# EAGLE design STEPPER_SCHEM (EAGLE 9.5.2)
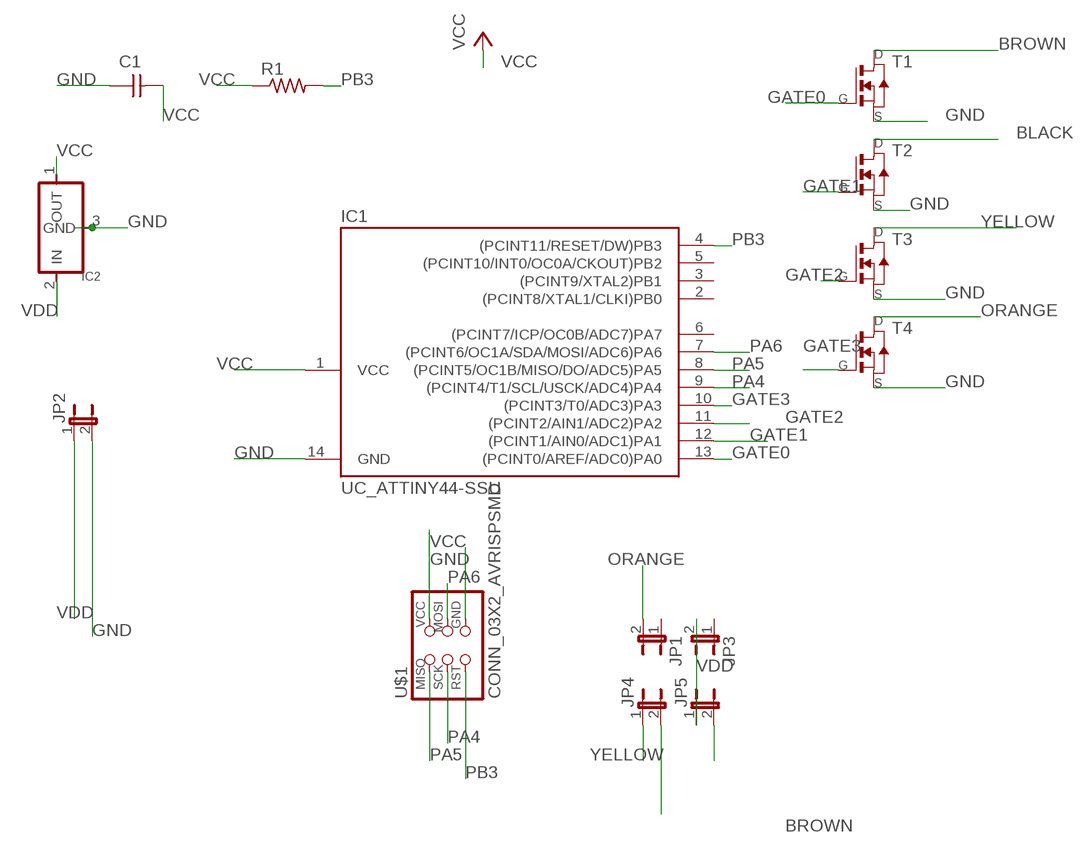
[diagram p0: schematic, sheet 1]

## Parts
C1  CAP_UNPOLARIZEDFAB  [C1206FAB]
IC1  UC_ATTINY44-SSU  [SOIC14]
IC2  VR_REGULATOR-SOT23SOT23  [SOT23]
JP1  JP1E  [JP1]
JP2  JP1E  [JP1]
JP3  JP1E  [JP1]
JP4  JP1E  [JP1]
JP5  JP1E  [JP1]
R1  R1206FAB  [R1206FAB]
T1  MOSFET_NSOT23  [SOT-23]
T2  MOSFET_NSOT23  [SOT-23]
T3  MOSFET_NSOT23  [SOT-23]
T4  MOSFET_NSOT23  [SOT-23]
U$1  CONN_03X2_AVRISPSMD  [2X03SMD]

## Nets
BLACK: JP4.2 T2.1(D)
BROWN: JP5.2 T1.1(D)
GATE0: IC1.13((PCINT0/AREF/ADC0)PA0) T1.3(G)
GATE1: IC1.12((PCINT1/AIN0/ADC1)PA1) T2.3(G)
GATE2: IC1.11((PCINT2/AIN1/ADC2)PA2) T3.3(G)
GATE3: IC1.10((PCINT3/T0/ADC3)PA3) T4.3(G)
GND: C1.1 IC1.14(GND) IC2.3(GND) JP2.2 T1.2(S) T2.2(S) T3.2(S) T4.2(S) U$1.6(GND)
ORANGE: JP1.2 T4.1(D)
PA4: IC1.9((PCINT4/T1/SCL/USCK/ADC4)PA4) U$1.3(SCK)
PA5: IC1.8((PCINT5/OC1B/MISO/DO/ADC5)PA5) U$1.1(MISO)
PA6: IC1.7((PCINT6/OC1A/SDA/MOSI/ADC6)PA6) U$1.4(MOSI)
PB3: IC1.4((PCINT11/RESET/DW)PB3) R1.2 U$1.5(RST)
VCC: C1.2 IC1.1(VCC) IC2.1(OUT) R1.1 U$1.2(VCC)
VDD: IC2.2(IN) JP2.1 JP3.2 JP5.1
YELLOW: JP4.1 T3.1(D)
Unconnected: IC1.2((PCINT8/XTAL1/CLKI)PB0) IC1.3((PCINT9/XTAL2)PB1) IC1.5((PCINT10/INT0/OC0A/CKOUT)PB2) IC1.6((PCINT7/ICP/OC0B/ADC7)PA7) JP1.1 JP3.1

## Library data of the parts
C1 = fab:CAP_UNPOLARIZED
IC1 = fab:UC_ATTINY44
IC2 = fab:VR_REGULATOR-SOT23
JP1-JP5 = jumper:JP1E: JUMPER
R1 = fab:R: Resistor (US Symbol)
T1-T4 = fab:MOSFET_N: MOS FET
U$1 = fab:CONN_03X2_AVRISP

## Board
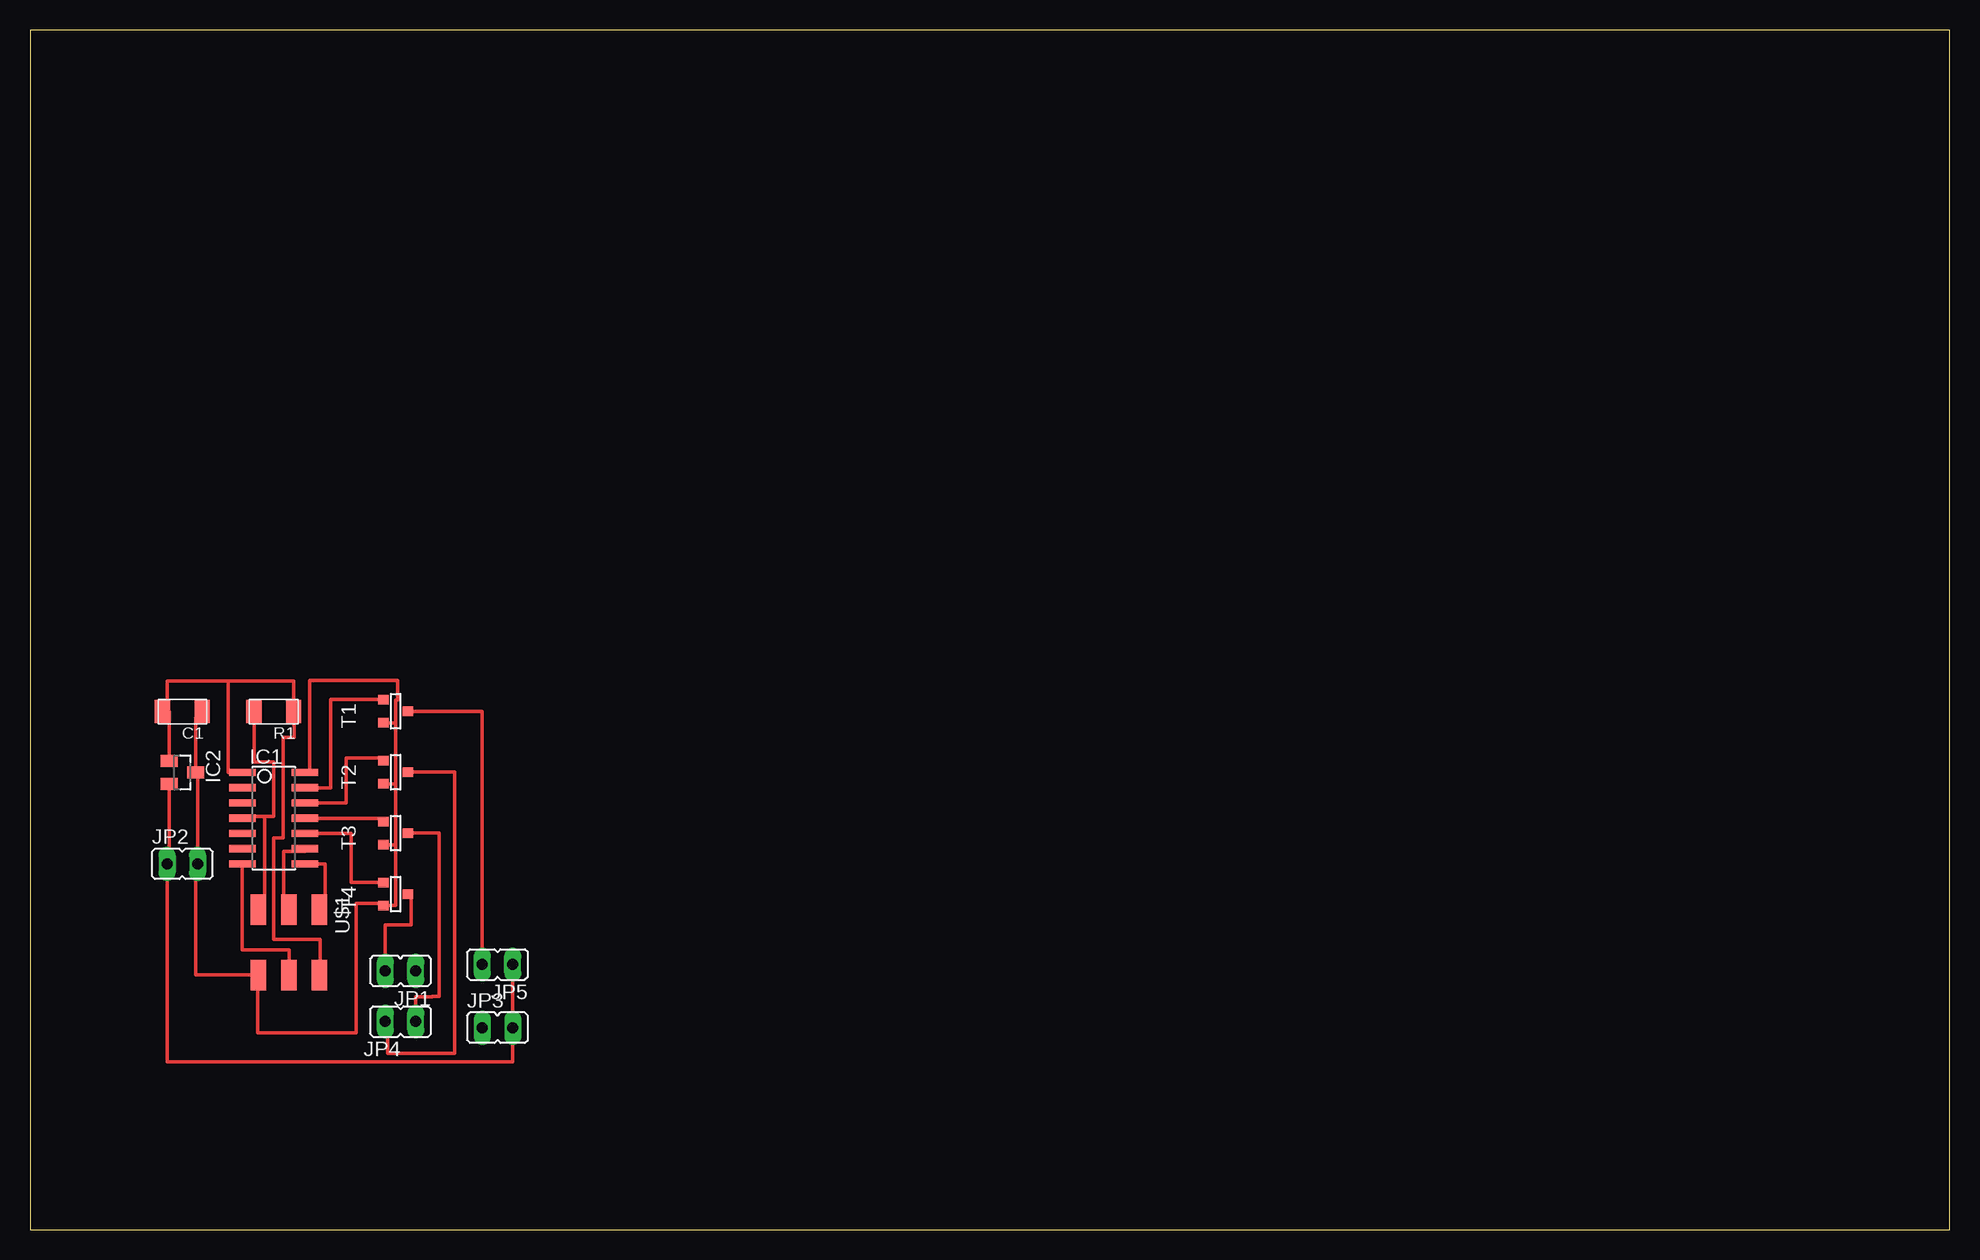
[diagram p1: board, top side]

Size 160 x 100 mm. Coordinates in mm from the lower left corner, seen from the top.
Outline: 0,0 160,0 160,100 0,100 0,0
Copper layers (1*16): Top 0.035mm / dielectric 0.15mm / Bottom 0.035mm
Design rules "default *": minimum track width 12mil, minimum drill 32mm, track to track 16mil, track to pad 16mil, pad to pad 16mil, via to via 16mil, smd to smd 16mil, copper to edge 16mil, drill to drill 16mil, minimum pad ring 10mil, minimum via ring 8mil, stop-mask expansion 4mil, vias tented up to drill 0mil, thermal gap 10mil

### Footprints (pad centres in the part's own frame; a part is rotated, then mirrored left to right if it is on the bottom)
C1206FAB = smd 1.27 x 1.905: 1 -1.651,0; 2 1.651,0
SOIC14 = smd 0.61 x 2.21: 1 -3.81,-2.603; 2 -2.54,-2.603; 3 -1.27,-2.603; 4 0,-2.603; 5 1.27,-2.603; 6 2.54,-2.603; 7 3.81,-2.603; 8 3.81,2.603; 9 2.54,2.603; 10 1.27,2.603; 11 0,2.603; 12 -1.27,2.603; 13 -2.54,2.603; 14 -3.81,2.603
SOT23 = smd 1 x 1.4: 1 -0.95,-1.1; 2 0.95,-1.1; 3 0,1.1
JP1 = drill 0.914 long: 1 0,-1.27; 2 0,1.27
R1206FAB = smd 1.27 x 1.905: 1 -1.651,0; 2 1.651,0
SOT-23 = smd 0.787 x 0.889: 1 0.025,-1.016; 2 -0.94,1.016; 3 0.991,1.016
2X03SMD = smd 2.54 x 1.27: 1 -2.54,2.54; 2 2.92,2.54; 3 -2.54,0; 4 2.92,0; 5 -2.54,-2.54; 6 2.92,-2.54

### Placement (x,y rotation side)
C1  12.7,43.18 180 top
IC1  20.32,34.29 270 top
IC2  12.7,38.1 270 top
JP1  30.89,21.56 90 top
JP2  12.7,30.48 270 top
JP3  38.96,16.81 270 top
JP4  30.89,17.35 90 top
JP5  38.96,22.1 90 top
R1  20.32,43.18 180 top
T1  30.48,43.18 90 top
T2  30.48,38.1 90 top
T3  30.48,33.02 90 top
T4  30.48,27.94 90 top
U$1  21.59,24.13 270 top

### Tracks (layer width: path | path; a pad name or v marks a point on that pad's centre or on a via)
BLACK
  Top 0.305: JP4.2 29.79,17.35 29.79,14.68 35.41,14.68 35.41,38.12 T2.1
BROWN
  Top 0.305: JP5.2 37.69,43.2 T1.1
GATE0
  Top 0.305: IC1.13 25.04,36.83 25.04,44.17 T1.3
GATE1
  Top 0.305: IC1.12 26.34,35.56 26.34,39.29 29.46,39.29 T2.3
GATE2
  Top 0.305: IC1.11 29.46,34.29 T3.3
GATE3
  Top 0.305: IC1.10 26.77,33.02 26.77,28.93 T4.3
GND
  Top 0.305: C1.1 13.8,42.63 IC2.3 13.97,38.1 13.97,30.66 | 13.97,30.66 JP2.2 | IC1.14 23.32,38.1 23.32,45.77 30.66,45.77 30.66,44.16 30.49,44.16 30.49,42.24 | 30.49,42.24 30.49,37.16 | 30.49,37.16 30.49,32.08 | 30.49,32.08 30.49,27 T4.2 29.46,27.2 27.2,27.2 27.2,16.41 19,16.41 19,21.21 U$1.6 13.82,21.21 13.82,30.66 13.97,30.66 | T1.2 30.49,42.24 | T2.2 30.49,37.16 | T3.2 30.49,32.08
ORANGE
  Top 0.305: T4.1 31.75,27.96 31.75,25.4 29.62,25.4 JP1.2
PA4
  Top 0.305: IC1.9 22.92,31.52 21.16,31.52 21.16,26.67 U$1.3
PA5
  Top 0.305: IC1.8 24.61,30.48 24.61,26.67 U$1.1
PA6
  Top 0.305: U$1.4 21.59,23.32 17.7,23.32 17.7,30.48 IC1.7
PB3
  Top 0.305: R1.2 18.67,38.96 20.32,38.96 20.32,34.42 19.56,34.42 | IC1.4 17.84,34.42 19.56,34.42 | 19.56,34.42 19.56,26.67 U$1.5
VCC
  Top 0.305: 11.43,39.22 IC2.1 11.6,43.18 C1.2 11.43,43.18 11.43,45.72 16.51,45.72 | 16.51,45.72 21.97,45.72 R1.1 22.02,43.18 22.02,41.02 21.11,41.02 21.11,32.64 20.3,32.64 20.3,24.18 24.18,24.18 24.18,21.21 U$1.2 | 16.51,45.72 16.51,38.1 IC1.1
VDD
  Top 0.305: JP3.2 JP5.1 40.23,13.97 11.66,13.97 11.43,13.97 JP2.1 11.6,30.48 IC2.2
YELLOW
  Top 0.305: JP4.1 32.16,19.38 33.53,19.38 33.53,19.43 34.11,19.43 34.11,33.05 T3.1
